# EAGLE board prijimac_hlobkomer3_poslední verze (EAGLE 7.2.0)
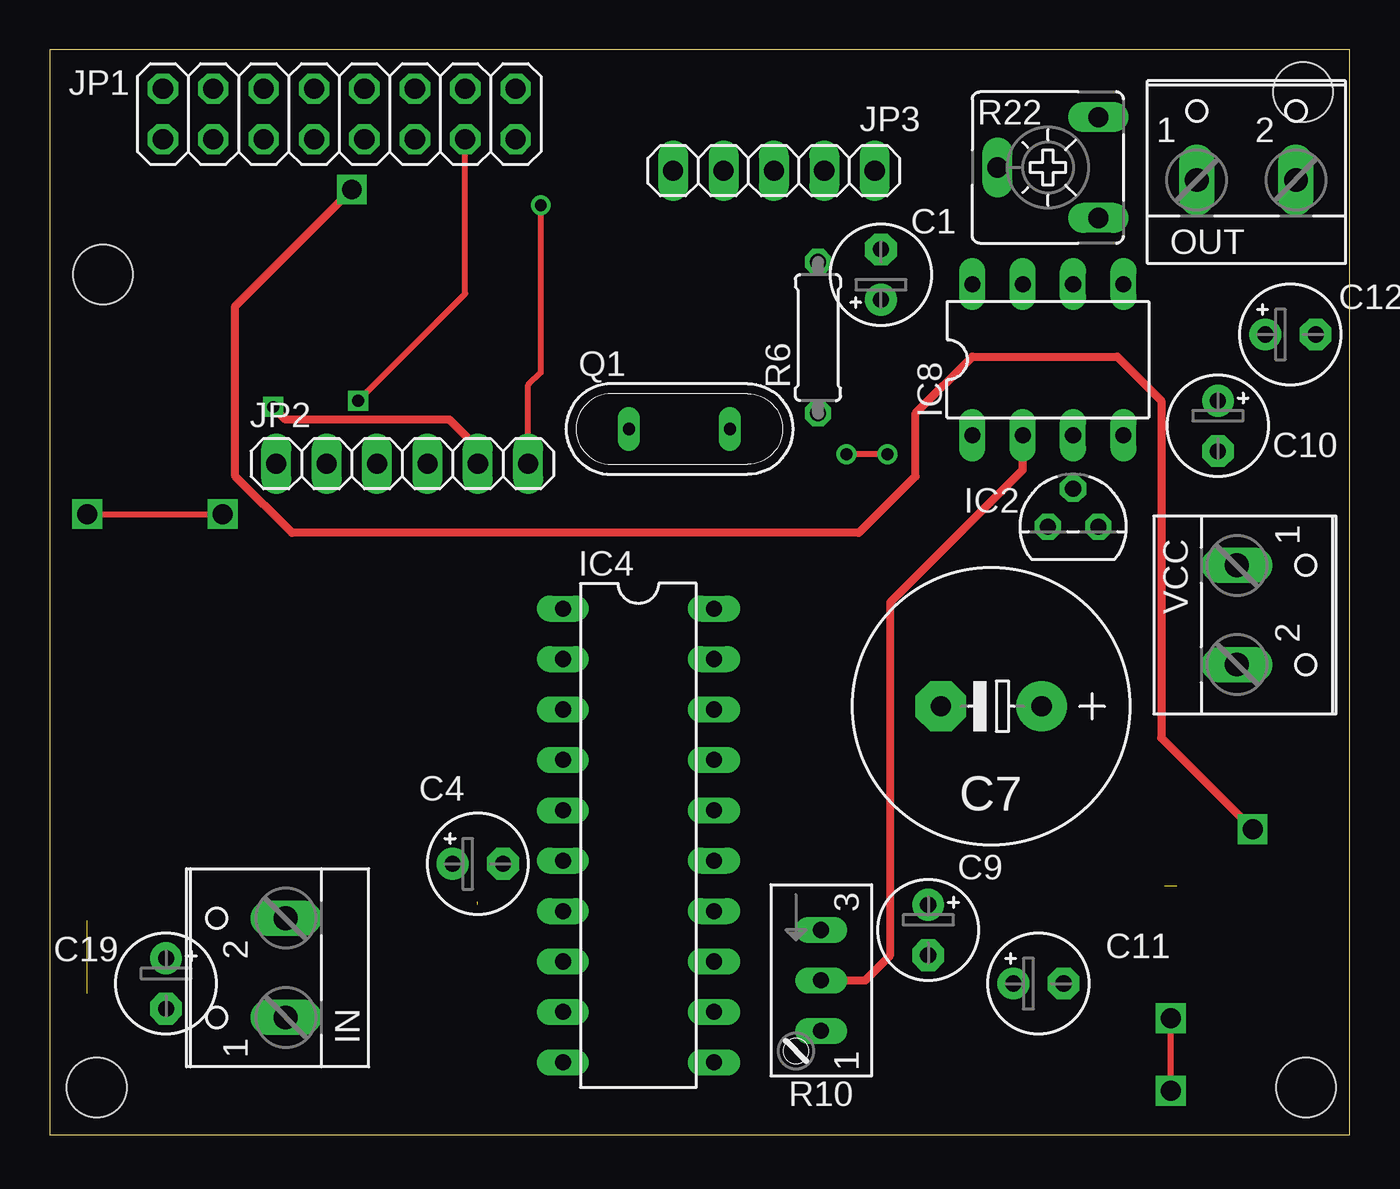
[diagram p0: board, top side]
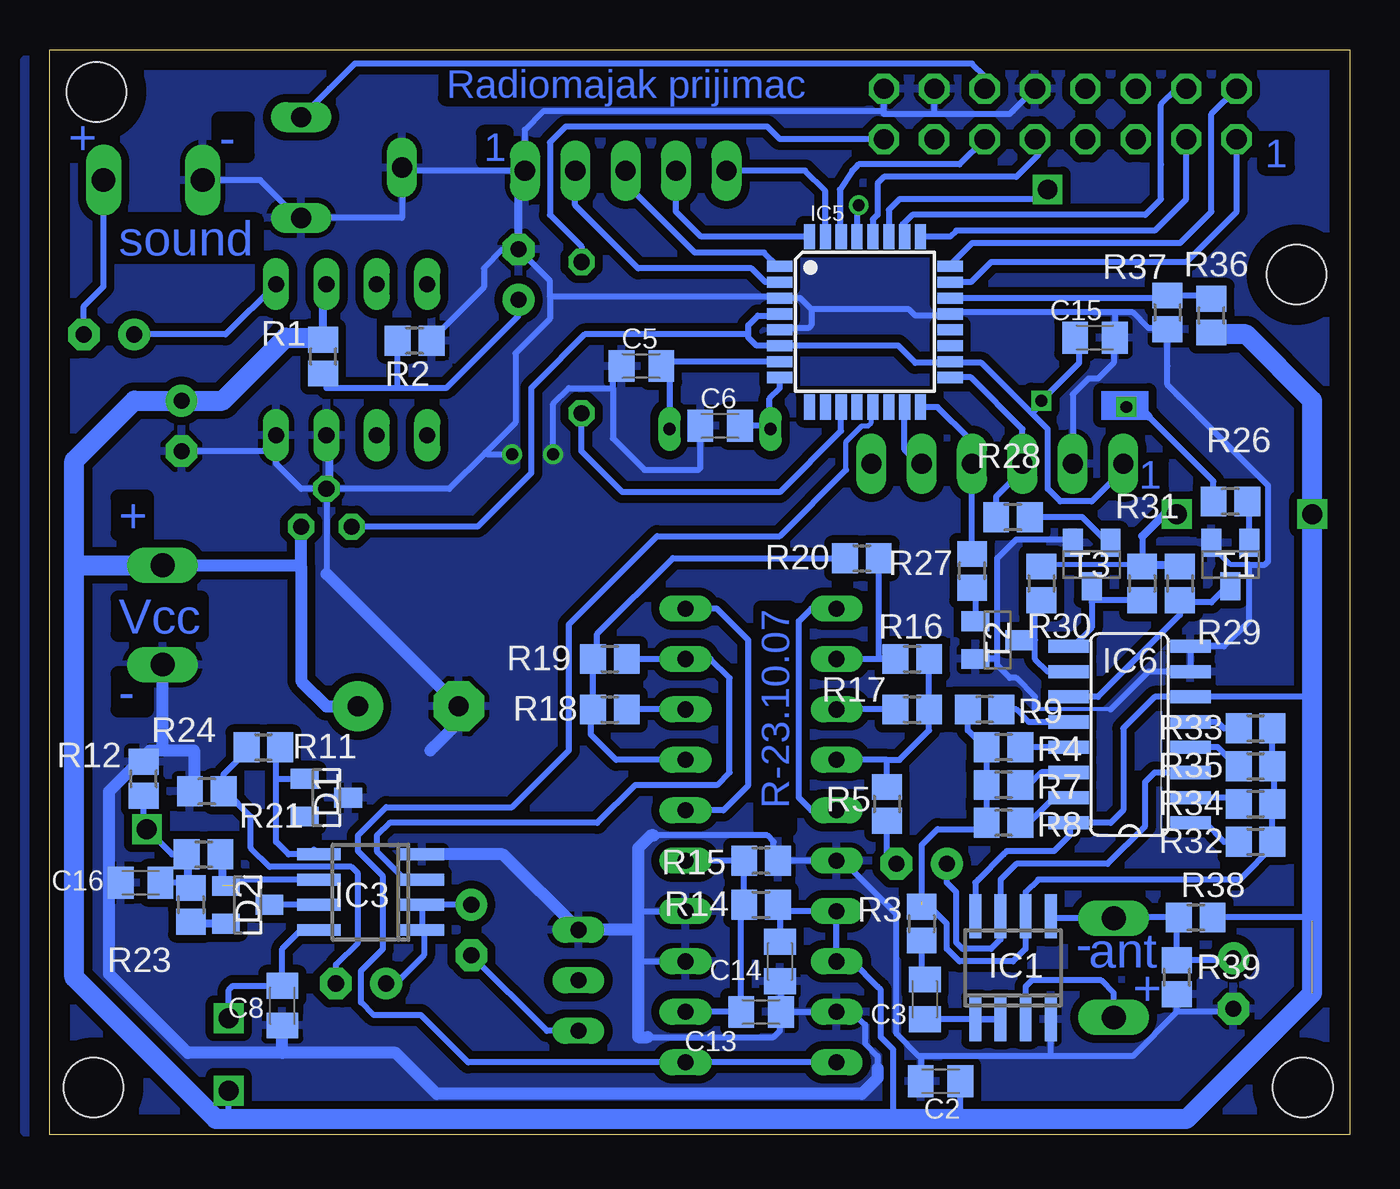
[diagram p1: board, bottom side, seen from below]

Size 65.54 x 54.67 mm. Coordinates in mm from the lower left corner, seen from the top.
Outline: 0,0 65.54,0 65.54,54.67 0,54.67 0,0
Copper layers (1*16): Top 0.035mm / dielectric 1.5mm / Bottom 0.035mm
Design rules "default": minimum track width 10mil, minimum drill 24mil, track to track 8mil, track to pad 8mil, pad to pad 8mil, via to via 8mil, smd to smd 8mil, copper to edge 40mil, drill to drill 8mil, minimum pad ring 10mil, minimum via ring 8mil, stop-mask expansion 4mil, vias tented up to drill 0mil, thermal gap 10mil
Holes 3 mm at 2.69,43.33 2.38,2.38 63.34,2.38 63.18,52.54

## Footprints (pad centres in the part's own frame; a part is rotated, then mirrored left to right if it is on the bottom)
E2,5-5 = drill 0.813 pad 1.6: + -1.27,0 | drill 0.813 pad 1.6 octagon: - 1.27,0
C0805K = smd 1.3 x 1.6: 1 -1,0; 2 1,0
E5-13 = drill 1.016 pad 2.54: + -2.54,0 | drill 1.016 pad 2.54 octagon: - 2.54,0
SOT23 = smd 1 x 1.4: 1 -0.95,-1.1; 2 0.95,-1.1; 3 0,1.1
SO08 = smd 0.6 x 2.2: 1 -1.905,-2.6; 2 -0.635,-2.6; 3 0.635,-2.6; 4 1.905,-2.6; 5 1.905,2.6; 6 0.635,2.6; 7 -0.635,2.6; 8 -1.905,2.6
TO92 = drill 0.813 octagon: 1 -1.27,0; 2 0,1.905; 3 1.27,0
DIL20 = drill 0.813 long: 1 -11.43,-3.81; 2 -8.89,-3.81; 3 -6.35,-3.81; 4 -3.81,-3.81; 5 -1.27,-3.81; 6 1.27,-3.81; 7 3.81,-3.81; 8 6.35,-3.81; 9 8.89,-3.81; 10 11.43,-3.81; 11 11.43,3.81; 12 8.89,3.81; 13 6.35,3.81; 14 3.81,3.81; 15 1.27,3.81; 16 -1.27,3.81; 17 -3.81,3.81; 18 -6.35,3.81; 19 -8.89,3.81; 20 -11.43,3.81
TQFP32-08 = smd 1.27 x 0.559: 1 -4.293,2.8; 2 -4.293,2; 3 -4.293,1.2; 4 -4.293,0.4; 5 -4.293,-0.4; 6 -4.293,-1.2; 7 -4.293,-2; 8 -4.293,-2.8; 17 4.293,-2.8; 18 4.293,-2; 19 4.293,-1.2; 20 4.293,-0.4; 21 4.293,0.4; 22 4.293,1.2; 23 4.293,2; 24 4.293,2.8 | smd 0.559 x 1.27: 9 -2.8,-4.293; 10 -2,-4.293; 11 -1.2,-4.293; 12 -0.4,-4.293; 13 0.4,-4.293; 14 1.2,-4.293; 15 2,-4.293; 16 2.8,-4.293; 25 2.8,4.293; 26 2,4.293; 27 1.2,4.293; 28 0.4,4.293; 29 -0.4,4.293; 30 -1.2,4.293; 31 -2,4.293; 32 -2.8,4.293
SO16 = smd 0.66 x 2.032: 1 -4.445,-3.073; 2 -3.175,-3.073; 3 -1.905,-3.073; 4 -0.635,-3.073; 5 0.635,-3.073; 6 1.905,-3.073; 7 3.175,-3.073; 8 4.445,-3.073; 9 4.445,3.073; 10 3.175,3.073; 11 1.905,3.073; 12 0.635,3.073; 13 -0.635,3.073; 14 -1.905,3.073; 15 -3.175,3.073; 16 -4.445,3.073
DIL08 = drill 0.813 long: 1 -3.81,-3.81; 2 -1.27,-3.81; 3 1.27,-3.81; 4 3.81,-3.81; 5 3.81,3.81; 6 1.27,3.81; 7 -1.27,3.81; 8 -3.81,3.81
W237-102 = drill 1.194 long: 1 -2.5,-1.27; 2 2.5,-1.27
2X08 = drill 1.016 octagon: 1 -8.89,-1.27; 2 -8.89,1.27; 3 -6.35,-1.27; 4 -6.35,1.27; 5 -3.81,-1.27; 6 -3.81,1.27; 7 -1.27,-1.27; 8 -1.27,1.27; 9 1.27,-1.27; 10 1.27,1.27; 11 3.81,-1.27; 12 3.81,1.27; 13 6.35,-1.27; 14 6.35,1.27; 15 8.89,-1.27; 16 8.89,1.27
1X06 = drill 1.016 long: 1 -6.35,0; 2 -3.81,0; 3 -1.27,0; 4 1.27,0; 5 3.81,0; 6 6.35,0
1X05 = drill 1.016 long: 1 -5.08,0; 2 -2.54,0; 3 0,0; 4 2.54,0; 5 5.08,0
QS = drill 0.61 long: 1 -2.54,0; 2 2.54,0
R0805 = smd 1.3 x 1.5: 1 -0.85,0; 2 0.85,0
0207/7 = drill 0.813 octagon: 1 -3.81,0; 2 3.81,0
S64W = drill 0.813 long: A 2.54,1.27; E -2.54,1.27; S 0,1.27
CA6V = drill 1.016 long: A -2.54,-2.54; E 2.54,-2.54; S 0,2.54
SOT23-BEC = smd 1 x 1.4: B -0.95,-1.1; C 0,1.1; E 0.95,-1.1

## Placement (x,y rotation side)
C1  10uF  [E2,5-5]  41.9,43.33 90 top
C2  100nF  [C0805K]  20.63,2.69 180 bottom
C3  100nF  [C0805K]  21.43,6.82 90 bottom
C4  10uF  [E2,5-5]  21.58,13.65 0 top
C5  12pF  [C0805K]  35.71,38.73 0 bottom
C6  33pF  [C0805K]  31.74,35.71 0 bottom
C7  2200uF/16V  [E5-13]  47.46,21.59 180 top
C8  100nF  [C0805K]  53.81,6.5 270 bottom
C9  10uF  [E2,5-5]  44.29,10.31 270 top
C10  100uF  [E2,5-5]  58.89,35.71 270 top
C11  10uF  [E2,5-5]  49.84,7.61 0 top
C12  100uF  [E2,5-5]  62.54,40.32 0 top
C13  100nF  [C0805K]  29.68,6.19 0 bottom
C14  100nF  [C0805K]  28.73,8.73 270 bottom
C15  100nF  [C0805K]  12.85,40.16 0 bottom
C16  100nF  [C0805K]  60.95,12.69 0 bottom
C19  10uF  [E2,5-5]  5.87,7.61 270 top
D1  BAS40-04  [SOT23]  51.59,16.98 270 bottom
D2  BAS40-04  [SOT23]  55.56,11.58 270 bottom
IC1  TL082D  [SO08]  16.98,8.41 0 bottom
IC2  78L05Z  [TO92]  51.59,30.63 0 top
IC3  LM358  [SO08]  49.37,12.22 90 bottom
IC4  [DIL20]  29.68,15.08 270 top
IC5  MEGA8-AI  [TQFP32-08]  24.44,40.95 0 bottom
IC6  4051D  [SO16]  11.11,20.16 90 bottom
IC8  LM384  [DIL08]  50.32,39.05 0 top
IN  [W237-102]  10.63,8.41 90 top
JP1  [2X08]  14.6,51.43 0 top
JP2  [1X06]  17.77,33.81 0 top
JP3  [1X05]  36.51,48.57 180 top
OUT  [W237-102]  60.32,49.37 0 top
Q1  [QS]  31.74,35.56 0 top
R1  10k  [R0805]  51.75,39.21 90 bottom
R2  10k  [R0805]  47.14,40 180 bottom
R3  10k  [R0805]  21.58,10.63 270 bottom
R4  2M2  [R0805]  17.46,19.52 180 bottom
R5  3k3  [R0805]  23.33,16.66 270 bottom
R6  47R  [0207/7]  38.73,40.16 90 top
R7  680k  [R0805]  17.46,17.62 180 bottom
R8  220k  [R0805]  17.46,15.71 180 bottom
R9  68k  [R0805]  18.41,21.43 180 bottom
R10  [S64W]  37.62,7.77 270 top
R11  220k  [R0805]  54.76,19.52 0 bottom
R12  220k  [R0805]  60.8,17.93 90 bottom
R14  1k  [R0805]  29.68,11.58 0 bottom
R15  1k  [R0805]  29.68,13.81 180 bottom
R16  100k  [R0805]  22.06,23.97 0 bottom
R17  2k  [R0805]  22.06,21.43 0 bottom
R18  2k  [R0805]  37.3,21.43 0 bottom
R19  100k  [R0805]  37.3,23.97 0 bottom
R20  3k3  [R0805]  24.6,29.05 0 bottom
R21  220k  [R0805]  57.78,14.12 0 bottom
R22  [CA6V]  50.32,48.73 90 top
R23  1k  [R0805]  58.41,11.58 270 bottom
R24  1k  [R0805]  57.62,17.3 180 bottom
R26  10k  [R0805]  6.03,31.9 180 bottom
R27  10k  [R0805]  19.04,28.41 90 bottom
R28  10k  [R0805]  16.98,31.11 180 bottom
R29  10k  [R0805]  8.57,27.78 270 bottom
R30  10k  [R0805]  15.55,27.78 270 bottom
R31  10k  [R0805]  10.47,27.78 270 bottom
R32  22k  [R0805]  4.76,14.76 0 bottom
R33  10k  [R0805]  4.76,20.47 0 bottom
R34  -  [R0805]  4.76,16.66 0 bottom
R35  -  [R0805]  4.76,18.57 0 bottom
R36  47k  [R0805]  6.98,41.27 90 bottom
R37  10k  [R0805]  9.2,41.43 270 bottom
R38  10k  [R0805]  7.77,10.95 0 bottom
R39  10k  [R0805]  8.73,7.93 90 bottom
T1  [SOT23-BEC]  6.03,28.73 180 bottom
T2  [SOT23-BEC]  17.77,24.92 270 bottom
T3  [SOT23-BEC]  13.01,28.73 180 bottom
VCC  [W237-102]  61.11,26.19 270 top

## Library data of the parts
C1-C16 C19 R1-R9 R11 R12 R14-R21 R23 R24 R26-R39 = rcl
D1 D2 = diode
IC1-IC3 IC8 = linear
IC4 = moje
IC5 = atmel
IC6 = 40xx
IN OUT VCC = con-wago-500
JP1-JP3 = pinhead
Q1 = special
R10 R22 = pot
T1-T3 = transistor

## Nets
0V: C1.+ R1.1 R2.2
+5V: C15.1 IC2.1 IC5.4 IC5.6 IC5.18 JP1.13 JP2.1
A: IC6.11 R29.2 T1.C
AGND: C19.+ IC1.5 IN.2 R38.1 R39.2
B: IC6.10 R30.2 T2.C
B$1-0: IC5.23 JP1.1
B$1-1: IC5.24 JP1.2
B$1-2: IC5.25 JP1.3
B$1-3: IC5.26 JP1.4
C: IC6.9 R31.2 T3.C
N$1: C3.2 R3.2
N$2: C4.- R5.2
N$3: C6.2 IC5.8 Q1.1
N$4: C3.1 IC1.1 IC1.2
N$5: C5.2 IC5.7 Q1.2
N$6: IC6.13 R4.1
N$7: IC1.6 R3.1 R4.2 R7.2 R8.2 R9.2 R32.2 R33.2 R34.2 R35.2
N$8: C4.+ IC1.7 IC6.3
N$9: IC6.14 R7.1
N$10: IC5.30 JP1.11
N$11: IC1.3 IN.1
N$12: IC6.15 R8.1
N$13: C13.1 IC4.12 IC4.15 R14.1 R15.2
N$14: C9.+ C11.+ IC3.1 IC3.2
N$15: C9.- R10.A
N$16: IC8.7
N$17: C11.- R11.1 R24.1
N$18: IC8.2 R10.S
N$19: C12.+ IC8.5
N$20: D1.1 IC3.5 R11.2
N$21: C12.- OUT.2
N$22: IC6.12 R9.1
N$23: IC4.1 IC4.5
N$24: IC4.16 IC4.20
N$25: IC4.4 R5.1 R16.2 R17.2
N$26: IC4.3 R17.1
N$27: IC4.2 R16.1 R20.2
N$28: IC3.3 IC4.19 R19.2
N$29: IC4.18 R18.2
N$30: IC4.17 R18.1 R19.1 R20.1
N$31: JP1.15 R6.2
N$32: IC5.11 R6.1
N$33: IC4.10 IC4.11 IC5.13
N$34: IC5.28 JP1.9
N$35: IC5.29 JP2.6
N$36: IC5.17 JP2.3 R28.2
N$37: IC5.16 JP2.4 R27.2
N$38: IC5.15 JP2.5 R26.2
N$39: D2.3 IC3.7
N$40: IC3.6 R21.2
N$41: IC5.22 R36.2 R37.1
N$42: JP1.12 R22.E
N$43: D2.2 R23.2
N$45: R26.1 T1.B
N$46: R27.1 T2.B
N$47: R28.1 T3.B
N$51: IC6.1 R32.1
N$52: IC6.5 R33.1
N$53: IC6.2 R34.1
N$54: IC6.4 R35.1
TL1: IC5.31 JP3.5
TL2: IC5.32 JP3.4
TL3: IC5.1 JP3.3
TL4: IC5.2 JP3.2
V+: C2.1 C7.+ C8.1 C10.+ C14.1 IC1.8 IC2.3 IC3.8 IC4.7 IC4.8 IC6.6 IC6.16 IC8.6 R1.2 R14.2 R29.1 R30.1 R31.1 R36.1 R38.2 VCC.1
V-: C1.- C2.2 C5.1 C6.1 C7.- C8.2 C10.- C13.2 C14.2 C15.2 C16.1 C19.- D1.3 IC1.4 IC2.2 IC3.4 IC4.6 IC4.9 IC4.13 IC4.14 IC5.3 IC5.5 IC5.21 IC6.7 IC6.8 IC8.3 IC8.4 JP1.10 JP1.14 JP1.16 JP2.2 JP3.1 OUT.1 R2.1 R10.E R12.2 R15.1 R22.A R22.S R24.2 R37.2 R39.1 T1.E T2.E T3.E VCC.2
VMER: C16.2 IC5.27 R12.1 R21.1 R23.1

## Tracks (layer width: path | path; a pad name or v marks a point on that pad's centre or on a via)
0V
  Bottom 0.305: C1.+ 41.9,41.27 45.55,37.62 48.09,37.62 | 48.09,37.62 51.59,37.62 51.59,38.25 51.75,38.41 R1.1 | R2.2 47.99,37.72 48.09,37.62
+5V  (via drill 0.6)
  Top 0.305: JP1.13 20.95,42.38 v15.55,36.98
  Bottom 0.305: 20.31,38.89 21.9,38.89 22.77,39.75 28.66,39.75 28.73,39.68 28.73,39.69 IC5.6 29.91,39.75 30.32,40.16 30.32,40.32 | JP2.1 11.42,33.49 13.01,31.9 14.6,31.9 15.23,32.54 15.23,35.56 16.03,36.35 | 16.03,36.35 18.57,38.89 20.31,38.89 | 20.31,38.89 20.25,38.95 IC5.18 | 40.95,37.94 38.57,40.32 30.32,40.32 | 16.03,36.35 15.55,36.83 v15.55,36.98 13.65,38.89 13.65,40 13.81,40.16 C15.1 | 30.32,40.32 30.32,40.79 29.84,41.27 28.73,41.27 28.73,41.28 IC5.4 | 30.32,40.32 | 40.95,37.94 | 40.95,37.94 41.27,37.62 41.27,33.33 43.97,30.63 IC2.1 | IC2.1
A
  Bottom 0.305: IC6.11 12.69,22.06 8.57,26.19 8.57,26.82 | 8.57,27.14 R29.2 8.57,26.82 | T1.C 6.17,27.63 6.98,26.82 8.57,26.82
AGND
  Bottom 0.305: 15.08,10.95 15.04,10.91 | C19.+ 5.97,8.78 R39.2 8.73,10.79 8.57,10.95 R38.1 11.9,10.95 IN.2 15.04,10.91 | 15.08,10.95 IC1.5 | 15.04,10.91 15.08,10.95
B
  Bottom 0.305: IC6.10 15.23,23.33 15.87,23.97 15.87,24.92 | R30.2 15.77,26.93 15.87,26.82 15.87,24.92 | 15.87,24.92 T2.C
B$1-0
  Bottom 0.305: IC5.23 19.11,42.95 18.09,43.97 8.25,43.97 5.71,46.51 5.71,49.68 5.87,49.84 5.71,50 JP1.1
B$1-1
  Bottom 0.305: JP1.2 6.98,51.43 6.98,46.51 8.57,44.92 19.04,44.92 20.16,43.81 20.15,43.8 IC5.24
B$1-2
  Bottom 0.305: IC5.25 20.15,45.25 19.84,45.56 9.84,45.56 8.25,47.14 8.25,50 8.41,50.16 JP1.3
B$1-3
  Bottom 0.305: JP1.4 8.73,52.7 9.52,51.91 9.52,48.89 | 10.31,46.35 22.06,46.35 22.54,45.87 22.54,45.24 22.53,45.25 IC5.26 | 10.31,46.35 | 10.31,46.35 9.52,47.14 9.52,48.89 | 9.52,48.89
C
  Bottom 0.305: IC6.9 13.96,24.6 13.01,25.55 13.01,26.82 | 13.01,26.82 T3.C | R31.2 12.91,26.93 13.01,26.82
N$1
  Bottom 0.305: 21.43,10 R3.2 21.58,8.09 21.43,7.93 C3.2
N$2
  Bottom 0.305: C4.- | R5.2 23.33,14.12 C4.-
N$3
  Bottom 0.305: 29.2,35.71 29.2,36.35 29.25,36.4 29.25,37.1 28.73,37.62 28.73,38.1 IC5.8 | Q1.1 29.2,35.71 | C6.2 29.2,35.71
N$4
  Bottom 0.305: IC1.1 18.89,5.87 18.82,5.81 IC1.2 21.05,5.81 21.43,5.87 C3.1
N$5
  Bottom 0.305: IC5.7 34.54,38.95 34.71,38.78 C5.2 34.44,38.73 34.28,38.89 Q1.2
N$6
  Bottom 0.305: IC6.13 R4.1
N$7  (1 unrouted)
  Bottom 0.305: R4.2 18.09,19.52 18.31,19.74 | R4.2 18.31,17.72 18.41,17.62 R7.2 18.31,15.61 | 18.31,15.61 R8.2 | 18.31,15.61 18.09,15.39 20.79,15.39 21.58,14.6 21.58,11.74 | 3.8,18.57 R35.2 | R33.2 3.91,18.67 3.8,18.57 | 3.8,18.57 3.8,16.66 R34.2 3.91,14.86 3.8,14.76 | 3.8,14.76 R32.2 4.12,14.76 | R4.2 18.41,19.52 19.26,20.37 R9.2 | 3.8,14.76 3.8,14.6 5.55,12.85 15.71,12.85 16.35,12.22 16.35,10.95 | 16.35,10.95 IC1.6 | R3.1 21.43,11.58 | 16.35,10.95 16.35,9.36 16.98,8.73 19.68,8.73 20.31,9.36 20.31,10.63 20.95,11.27 21.27,11.27 21.58,11.58 R3.1 | R3.1 21.16,11.48
N$8
  Bottom 0.305: IC6.3 9.84,18.25 10.31,17.78 10.31,15.55 12.22,13.65 16.82,13.65 17.62,12.85 IC1.7 17.62,9.84 18.09,9.36 19.52,9.36 19.84,9.68 19.84,12.22 20.31,12.7 C4.+
N$9
  Bottom 0.305: IC6.14 15.55,18.25 16.19,17.62 R7.1
N$10
  Bottom 0.305: IC5.30 25.71,45.25 25.71,45.24 25.71,47.62 25.08,48.57 | 25.08,48.57 | 24.92,48.73 25.08,48.57 | 24.92,48.73 | 24.92,48.73 24.76,48.89 19.68,48.89 JP1.11 | JP1.11
N$11
  Bottom 0.305: 16.35,5.87 IC1.3 16.35,7.46 16.03,7.77 12.54,7.77 11.9,7.14 IN.1 11.9,5.87
N$12
  Bottom 0.305: R8.1 16.19,15.71 14.92,16.98 IC6.15 13.96,16.98
N$13
  Bottom 0.305: R15.2 30.32,13.81 | R15.2 IC4.15 | R15.2 30.53,11.69 30.63,11.58 | C13.1 30.63,6.19 | C13.1 IC4.12 | 30.63,11.58 R14.1 | C13.1 30.68,11.54 30.63,11.58
N$14
  Bottom 0.305: C9.+ IC3.2 46.83,11.58 46.77,11.52 IC3.1 46.67,10.31 46.67,9.04 48.09,7.62 C11.+
N$15
  Bottom 0.305: R10.A 40.48,5.23 C9.-
N$17
  Bottom 0.305: C11.- 51.11,8.57 50,9.68 50,13.17 50.32,13.49 54.45,13.49 55.4,14.44 55.4,16.03 56.67,17.3 | 56.67,17.3 | 56.67,17.3 R24.1 56.77,18.15 55.4,19.52 R11.1
N$18
  Top 0.406: R10.S 41.11,7.77 42.38,9.04 42.38,26.82 49.05,33.49 IC8.2
N$19
  Bottom 0.305: C12.+ 56.67,40.32 IC8.5
N$20
  Bottom 0.305: IC3.5 52.22,14.38 52.22,14.12 53.49,14.12 54.13,14.76 54.13,17.93 | R11.2 53.81,19.52 54.13,19.2 54.13,17.93 | D1.1 54.12,17.93 54.13,17.93
N$21
  Bottom 0.305: OUT.2 62.82,42.74 63.81,41.75 63.81,40.48 63.97,40.32 C12.-
N$22
  Bottom 0.305: IC6.12 16.19,20.79 16.82,21.43 R9.1 17.77,21.43
N$23
  Bottom 0.305: IC4.1 27.14,26.51 27.78,25.87 27.78,16.98 27.14,16.35 IC4.5
N$24
  Bottom 0.305: IC4.20 31.9,26.51 30.32,24.92 30.32,17.62 31.59,16.35 IC4.16
N$25
  Bottom 0.305: R16.2 21.21,21.53 21.11,21.43 R17.2 21.21,20.37 22.7,18.89 23.33,18.89 | 23.33,18.89 IC4.4 | R5.1 23.33,18.89
N$26
  Bottom 0.305: R17.1 IC4.3
N$27
  Bottom 0.305: 22.7,23.97 R16.1 23.65,23.97 | 23.65,23.97 IC4.2 | R20.2 23.75,24.07 23.65,23.97
N$28
  Bottom 0.305: 36.66,23.97 R19.2 IC4.19 32.22,23.97 31.27,23.01 31.27,18.25 31.9,17.62 36.03,17.62 37.94,15.71 48.41,15.71 49.05,15.08 49.05,14.28 47.62,12.85 IC3.3
N$29
  Bottom 0.305: IC4.18 R18.2
N$30
  Bottom 0.305: IC4.17 36.98,18.89 38.25,20.16 38.25,21.43 R18.1 38.15,23.86 38.25,23.97 | 38.25,23.97 R19.1 | 38.25,23.97 37.94,24.28 37.94,25.24 34.12,29.05 25.55,29.05 25.45,29.15 | 25.45,29.15 25.39,29.21 | 25.45,29.15 R20.1
N$31
  Bottom 0.305: R6.2 38.73,44.76 40.16,46.19 40.32,46.35 40.32,50 39.52,50.8 29.36,50.8 28.73,50.16 23.65,50.16 23.49,50 | JP1.15 | 23.49,50 | JP1.15 23.49,50
N$32
  Bottom 0.305: 28.73,32.38 36.66,32.38 38.73,34.44 R6.1 | IC5.11 25.64,35.47 28.73,32.38 | 28.73,32.38
N$33
  Bottom 0.254: 25.39,33.49 25.39,34.92 24.76,35.56 | 24.76,35.56 | 24.76,35.56 24.6,35.71 24.28,35.71 24.12,35.87 24.12,36.67 24.12,36.66 IC5.13
  Bottom 0.305: 24.12,36.83 24.04,36.74 IC5.13 | IC4.10 IC4.11 44.44,3.65 46.83,6.03 49.21,6.03 49.84,6.66 49.84,8.25 48.73,9.36 48.73,13.01 50,14.28 50,15.08 48.57,16.51 42.22,16.51 39.36,19.36 39.36,25.71 34.92,30.16 28.73,30.16 25.39,33.49
N$34
  Bottom 0.305: JP1.9 15.87,50 15.71,49.84 15.71,49.37 16.82,48.26 23.49,48.26 23.81,47.94 23.81,46.35 23.96,46.19 | IC5.28 24.04,46.12 23.96,46.19 | 23.96,46.19
N$35  (via drill 0.6)
  Top 0.305: v24.76,46.83 24.76,38.41 24.12,37.78 JP2.6
  Bottom 0.305: IC5.29 24.84,46.74 v24.76,46.83
N$36
  Bottom 0.305: IC5.17 19.1,38.15 16.5,35.56 JP2.3 16.5,33.49 16.66,33.33 | 16.66,33.33 | R28.2 17.83,32.17 16.66,33.33
N$37
  Bottom 0.305: IC5.16 20.78,36.66 19.2,35.08 19.2,33.49 JP2.4 19.04,29.36 19.15,29.26 | 19.15,29.26 19.2,29.21 | R27.2 19.15,29.26
N$38  (via drill 0.6)
  Top 0.406: JP2.5 21.58,34.6 20.16,36.03 11.9,36.03 v11.27,36.67
  Bottom 0.305: JP2.5 21.58,33.65 22.44,34.51 IC5.15 22.38,36.66 22.38,36.67 | R26.2 6.88,32.91 10.15,36.19
  Bottom 0.406: v11.27,36.67 10.63,36.67 10.15,36.19
N$39
  Bottom 0.305: 54.6,11.58 D2.3 IC3.7
N$40  (1 unrouted)
  Bottom 0.305: 56.19,12.53 56.19,12.85 IC3.6
  Bottom 0.406: R21.2 56.83,14.12 56.83,12.53
N$41
  Bottom 0.305: 20.24,42.15 20.31,42.22 | 20.24,42.15 IC5.22 9.29,42.15 9.2,42.06 R37.1 7.04,42.28 6.88,42.12 | 20.24,42.15 20.21,42.12 | 6.88,42.12 6.82,42.06 | R36.2 6.88,42.12
N$42
  Bottom 0.305: 51.43,52.7 R22.E | JP1.12 18.41,53.34 19.04,53.97 50.16,53.97 51.43,52.7 | 51.43,52.7
N$43
  Bottom 0.406: 58.57,10.63 58.57,10.73 R23.2 | D2.2 58.57,10.63 | 58.57,10.63
N$45
  Bottom 0.305: 5.08,32.22 5.18,32.12 R26.1 | T1.B 5.08,32.22 | 5.08,32.22 5.07,32.22
N$46
  Bottom 0.305: R27.1 19.04,27.78 18.87,27.61 T2.B
N$47
  Bottom 0.305: T3.B 12.21,29.83 13.49,31.11 R28.1
N$51
  Bottom 0.305: IC6.1 7.3,15.71 6.34,14.76 R32.1 5.39,14.76
N$52
  Bottom 0.305: R33.1 6.34,20.47 6.66,20.79 IC6.5 8.25,20.79
N$53
  Bottom 0.305: 8.25,16.98 IC6.2 6.03,16.98 5.71,16.66 R34.1
N$54
  Bottom 0.305: IC6.4 6.66,19.52 5.71,18.57 R35.1
TL1
  Bottom 0.305: IC5.31 26.44,47.56 27.46,48.57 JP3.5 | JP3.5
TL2
  Bottom 0.305: IC5.32 32.7,45.25 33.97,46.51 JP3.4 33.97,48.73
TL3
  Bottom 0.305: JP3.3 36.51,47.94 33.01,44.45 29.52,44.45 28.83,43.75 IC5.1
TL4
  Bottom 0.305: IC5.2 29.46,42.95 30.16,43.65 35.87,43.65 39.05,46.83 JP3.2
V+  (via drill 1)  (1 unrouted)
  Top 0.305: v1.9,31.27 v8.73,31.27 | v56.51,2.22 v56.51,5.87
  Bottom 0.254: 15.55,28.73 | 15.55,28.73 R30.1 | 11.11,28.73 15.55,28.73
  Bottom 0.305: C14.1 28.73,11.58 R14.2 28.83,11.37 28.73,11.27 IC4.7 IC4.8 25.08,8.73 23.81,7.46 | IC3.8 52.22,10.31 | IC3.8 51.91,10.31 | IC3.8 52.86,10.31 53.81,9.36 C8.1 56.3,7.5 56.51,7.3 v56.51,5.87 | 8.57,28.41 R29.1 | 8.57,28.41 8.78,28.63 | 11.11,28.73 11,28.63 R31.1 10.47,30.16 | 15.55,28.73 R30.1 15.61,28.63 15.71,28.73 | 17.46,14.12 18.73,12.85 | 17.46,14.12 | 17.46,14.12 17.3,14.28 14.92,14.28 14.12,15.08 14.12,15.87 14.18,15.81 IC6.16 12.06,15.71 11.42,16.35 11.42,20.47 9.84,22.06 IC6.6 1.9,22.06 | 18.73,12.85 | 18.73,12.85 18.89,12.7 IC1.8 18.89,10.95 | R38.2 2.06,10.95 1.9,10.79 | 23.81,7.46 | 23.81,7.46 23.65,7.3 23.65,4.92 23.01,4.28 23.01,0.79 | C2.1 19.63,1.15 19.68,1.11 19.68,0.95 19.84,0.79 | 56.67,0.79 56.67,0.63 56.51,0.79 v56.51,2.22 | 8.57,28.41 8.73,28.41 9.04,28.73
  Bottom 0.406: 51.75,40.16 51.75,42.7 IC8.6 | R31.1 10.31,28.63 10.31,28.73 9.04,28.73 | v8.73,31.27 9.36,31.27 10.47,30.16
  Bottom 0.61: C7.+ 51.59,21.59 52.86,22.86 52.86,28.57 | 52.86,28.57 IC2.3 52.7,30.79 | VCC.1 52.98,28.69 52.86,28.57
  Bottom 1.016: VCC.1 64.25,28.69 64.29,28.73 | 64.29,28.73 64.29,7.93 57.14,0.79 56.67,0.79 56.51,0.79 23.01,0.79 19.84,0.79 8.25,0.79 1.9,7.14 1.9,22.06 v1.9,31.27 1.9,36.98 5.23,40.32 6.98,40.32 R36.1 | 64.29,28.73 64.29,33.97 61.27,36.98 C10.+ 56.83,36.98 53.65,40.16 51.75,40.16 R1.2
V-  (via drill 0.6)
  Top 0.305: v42.22,34.29 v40.16,34.29
  Bottom 0.2: 12.06,21.43 15.87,21.43
  Bottom 0.254: 6.98,29.68 6.03,28.73 5.07,28.73
  Bottom 0.305: 35.08,15.08 29.36,15.08 29.05,14.76 29.05,13.81 R15.1 28.83,13.7 | C14.2 28.73,7.77 28.68,7.73 C13.2 | C13.2 IC4.9 25.08,6.19 24.44,5.55 24.44,4.6 23.81,3.96 23.81,3.33 | C13.2 28.73,6.19 28.73,5.23 29.05,4.92 35.4,4.92 | 15.08,5.87 IC1.4 15.08,3.96 | IC3.4 46.83,14.12 | 7.93,24.6 8.03,24.5 IC6.7 10.15,23.33 12.06,21.43 | 6.98,29.68 T1.E 6.98,29.68 | 7.93,24.6 IC6.8 | 7.93,24.6 6.34,24.6 5.07,25.87 5.07,28.73 4.28,28.73 4.12,28.89 4.12,32.7 8.73,37.3 | 17.77,23.97 17.78,23.97 T2.E 19.2,23.97 | 17.77,23.97 17.77,23.65 17.14,23.01 16.82,23.01 15.87,22.06 15.87,21.43 | 17.77,23.97 17.77,29.05 16.82,30 13.96,30 T3.E 13.96,29.84 | 20.31,41.27 20.23,41.35 IC5.21 | IC5.21 20.15,41.42 20.16,41.43 11.9,41.43 | IC5.21 20.24,41.35 20.31,41.43 20.47,41.27 21.9,41.27 | JP1.10 | 16.98,51.59 JP1.10 | 16.98,51.59 | 16.98,51.59 17.14,51.43 20.95,51.43 | 20.95,51.43 23.49,51.43 23.49,51.59 | 23.49,51.59 JP1.16 | 20.95,51.43 JP1.14 | IC2.2 51.75,32.54 | 47.78,48.57 | 47.78,48.57 R22.S 47.78,46.19 | 47.78,48.57 JP3.1 41.43,48.57 | 47.78,46.19 | 47.78,46.19 R22.A 52.86,46.03 | 47.78,46.19 | 51.75,32.54 IC2.2 | 51.75,32.54 51.79,32.59 | 41.43,48.57 | 41.43,48.57 41.59,48.73 41.59,50.64 40.63,51.59 23.49,51.59 | 15.08,3.96 10.95,3.96 8.73,6.19 | C19.- 6.03,6.35 6.18,6.19 8.73,6.19 | 8.73,6.19 R39.1 | 28.83,13.7 28.89,13.65 | 28.83,13.7 28.73,13.81 IC4.6 25.39,13.81 25.39,13.65 22.85,11.11 22.85,5.08 21.74,3.96 21.58,3.96 | 21.9,41.27 | 21.9,41.27 22.22,41.59 | IC2.2 51.59,28.25 51.59,28.09 | 62.54,17.3 62.66,17.3 | 62.54,17.3 | 52.86,46.03 | OUT.1 54.92,48.1 52.86,46.03 | 54.13,35.08 IC8.4 | C10.- 54.76,34.44 54.13,35.08 | 54.13,35.08 54.13,33.81 52.86,32.54 51.43,32.54
  Bottom 0.305: 51.43,32.54 IC2.2 | R2.1 46.29,40.06 43.65,42.7 43.65,43.65 42.7,44.6 C1.- | VCC.2 59.96,23.69 | R24.2 58.47,17.4 58.26,17.62 | 51.43,32.54 45.4,32.54 43.57,34.36 | 43.57,34.36 42.06,35.87 42.06,39.37 40.32,41.11 40.32,42.22 | 15.08,3.96 21.58,3.96 | C2.2 21.63,3.92 21.58,3.96 | 8.73,37.3 9.2,37.78 9.2,38.73 | 8.73,37.3 8.57,37.14 | 23.49,51.59 | 11.9,41.43 10.95,41.43 10.15,40.64 9.04,40.64 9.1,40.58 R37.2 9.2,38.73 | 9.2,38.73 | JP2.2 13.96,37.3 13.17,38.1 12.69,38.1 11.9,38.89 11.9,40 11.85,40.05 C15.2 11.85,41.38 11.9,41.43 | 27.14,41.59 27.71,42.15 IC5.3 28.66,42.15 | 27.14,41.59 27.14,40.79 27.3,40.64 28.41,40.64 28.57,40.48 28.64,40.55 IC5.5 | 22.22,41.59 | 22.22,41.59 27.14,41.59 | v40.16,34.29 40.16,36.83 39.36,37.62 37.14,37.62 | 43.57,34.36 43.49,34.29 v42.22,34.29 | C6.1 32.74,33.6 32.86,33.49 35.55,33.49 37.14,35.08 37.14,37.62 | 37.14,37.62 37.14,38.41 36.82,38.41 36.66,38.57 36.71,38.62 C5.1 | 28.66,42.15 28.57,42.06 | 28.66,42.15 28.73,42.22 40.32,42.22 | C1.- | 40.32,42.22 40.32,43.02 C1.- | 62.7,12.7 | 62.38,12.7 62.7,12.7 | 62.7,12.7 | 35.87,11.27 IC4.14 | 35.87,8.73 IC4.13
  Bottom 0.406: JP3.1 41.9,48.57 C1.- | IC2.2 51.43,32.54 51.43,35.24 IC8.3
  Bottom 0.61: 51.59,28.25 45.24,21.9 45.24,20.47 46.19,19.52 | 46.19,19.52 | 46.19,19.52 46.35,19.36 | 59.84,19.36 58.26,19.36 58.26,17.62 | 59.84,19.36 60.48,19.36 62.54,17.3 62.54,8.09 58.57,4.12 53.81,4.12 | 59.84,19.36 VCC.2 | C16.1 62.38,12.7 | 53.81,4.12 48.09,4.12 46.03,2.06 24.6,2.06 23.81,2.85 23.81,3.33 | 53.81,4.12 C8.2 | 35.4,4.92 35.87,4.92 35.87,8.73 35.87,10.31 | 35.08,15.08 35.24,15.08 35.87,14.44 35.87,11.27 35.87,10.31 | 35.87,10.31 R10.E 42.7,14.12 IC3.4
  pour Bottom (isolate 0.406): -0.48,55.4 -0.48,-0.8 -0.17,-1.12 65.56,-1.12 66.83,0.15 66.83,54.13 65.24,55.72 -0.17,55.72
VMER  (via drill 1)
  Top 0.406: v60.64,15.39 56.03,20 56.03,36.98 53.81,39.21 46.51,39.21 43.65,36.35 43.65,33.17 40.79,30.32 12.22,30.32 9.36,33.17 9.36,41.75 v15.23,47.62
  Bottom 0.305: R23.1 | C16.2 58.41,12.7 R23.1 | IC5.27 23.24,46.6 22.7,47.14 15.71,47.14 v15.23,47.62 | R21.1 59.37,14.12 v60.64,15.39 60.8,15.39 R12.1
  Bottom 0.406: R21.1 58.57,14.12 58.57,12.43 R23.1
(copper drawn outside any net)
  shapes: Bottom area x1

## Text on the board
Bottom: Radiomajak prijimac | - | + | 1 | 1 | sound | 1 | + | R-23.10.07 | Vcc | - | ant | - | +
